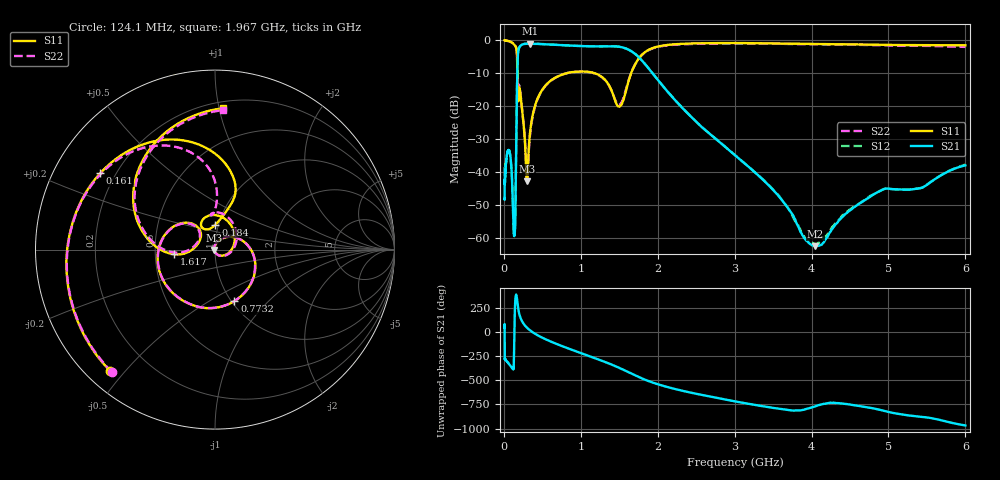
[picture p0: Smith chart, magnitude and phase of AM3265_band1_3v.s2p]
!Agilent Technologies,E8364B,MY43040894,A.07.50.67
!Agilent E8364B: A.07.50.67
!Date: Friday, May 09, 2025 07:14:46
!Correction: S11(Full 2 Port(1,2))
!S21(Full 2 Port(1,2))
!S12(Full 2 Port(1,2))
!S22(Full 2 Port(1,2))
!S2P File: Measurements: S11, S21, S12, S22:Log Frequency Sweep
# Hz S  dB  R 50
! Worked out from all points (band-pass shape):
!   3201 points, 10 MHz to 6 GHz, reference 50 ohm
!   highest |S21| = -0.99 dB at 335.9 MHz (marker M1); lowest = -62.6 dB at 4.047 GHz (marker M2)
!   |S21| within 3 dB of the highest: 183.9 MHz to 1.701 GHz (1.517 GHz wide, 161 % of centre)
!   lowest |S11| = -42.9 dB at 301 MHz (marker M3), VSWR 1.01, Z = 49.3 - j0.177 ohm
!   |S11| at or under -10 dB: 176 MHz to 810.6 MHz (634.6 MHz wide, 129 % of centre); 1.185 GHz to 1.654 GHz (469.7 MHz wide, 33.1 % of centre)
!   |S22| runs from -41.4 to 0.0 dB; largest |S21 - S12| = 0.014
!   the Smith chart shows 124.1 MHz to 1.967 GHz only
!   S11 on the Smith chart (normalised r, x): 124.1 MHz: 0.07, -0.45; 161 MHz: 0.14, +0.30; 184 MHz: 0.97, +0.27; 773.2 MHz: 1.03, -0.65; 1.617 GHz: 0.63, -0.03; 1.967 GHz: 0.25, +1.03
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1e7  -0.02 -9.0  -48.11 44.4  -38.51 64.8  -0.11 -8.6
2.908064e7  -0.06 -25.3  -36.89 65.6  -36.96 65.2  -0.06 -25.4
8.439949e7  -0.35 -79.1  -35.14 10.8  -35.11 10.4  -0.39 -79.1
1.241358e8  -0.98 -130.9  -55.59 -23.5  -55.85 73.3  -1.00 -130.0
1.453726e8  -1.54 -170.2  -57.36 -67.7  -55.90 -48.0  -1.52 -167.7
1.609754e8  -2.29 146.4  -30.94 25.5  -31.00 25.8  -2.21 152.3
1.840463e8  -17.13 89.0  -3.95 -100.5  -3.91 -100.4  -12.78 89.4
2.050257e8  -14.55 80.5  -1.98 173.9  -1.94 173.9  -14.13 70.6
2.44949e8  -22.76 -19.3  -1.18 100.4  -1.15 100.4  -22.47 -21.4
3.009521e8  -42.87 -165.5  -1.01 44.7  -0.97 44.7  -41.32 -160.8
3.359285e8  -29.12 78.3  -0.99 20.2  -0.96 20.2  -29.72 85.0
7.123273e8  -10.82 -52.6  -1.39 -132.1  -1.36 -132.1  -10.83 -53.1
7.731694e8  -10.26 -69.4  -1.47 -151.0  -1.43 -151.0  -10.27 -70.0
1.188315e9  -10.03 179.9  -1.80 87.7  -1.77 87.8  -10.10 179.0
1.616703e9  -12.72 -173.6  -2.76 -54.5  -2.73 -54.5  -12.49 -176.4
1.966578e9  -2.06 86.8  -10.96 -172.1  -10.94 -172.0  -2.18 86.8
2.067357e9  -1.55 62.8  -13.86 163.2  -13.84 163.3  -1.68 63.1
2.455151e9  -0.91 -11.0  -23.69 87.7  -23.64 87.7  -1.05 -10.4
2.96862e9  -0.79 -90.1  -34.16 7.0  -34.13 7.0  -0.90 -90.3
4.046889e9  -1.06 124.3  -62.55 -50.2  -61.93 -54.3  -1.17 121.8
5.002045e9  -1.35 4.4  -45.06 -108.7  -45.15 -108.7  -1.53 4.8
6e9  -1.46 -115.1  -37.98 112.3  -37.76 111.4  -1.96 -110.9
